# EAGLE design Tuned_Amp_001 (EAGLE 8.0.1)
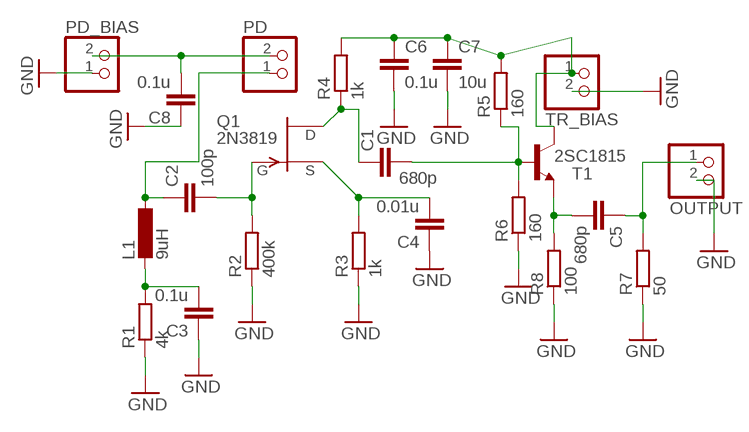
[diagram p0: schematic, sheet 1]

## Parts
C1  680p  C-EU025-024X044  [C025-024X044]
C2  100p  C-EU025-024X044  [C025-024X044]
C3  0.1u  C-EU025-024X044  [C025-024X044]
C4  0.01u  C-EU025-024X044  [C025-024X044]
C5  680p  C-EU025-024X044  [C025-024X044]
C6  0.1u  C-EU025-024X044  [C025-024X044]
C7  10u  C-EU025-024X044  [C025-024X044]
C8  0.1u  C-EU025-024X044  [C025-024X044]
L1  9uH  L-EU0207/10  [0207/10]
OUTPUT  JST_2PIN-SMT  [JST-PH-2-SMT]
PD  JST_2PIN-SMT  [JST-PH-2-SMT]
PD_BIAS  JST_2PIN-SMT  [JST-PH-2-SMT]
Q1  2N3819  [TO92]
R1  4k  R-EU_0207/10  [0207/10]
R2  400k  R-EU_0207/10  [0207/10]
R3  1k  R-EU_0207/10  [0207/10]
R4  1k  R-EU_0207/10  [0207/10]
R5  160  R-EU_0207/10  [0207/10]
R6  160  R-EU_0207/10  [0207/10]
R7  50  R-EU_0207/10  [0207/10]
R8  100  R-EU_0207/10  [0207/10]
T1  2SC1815  [TO92-ECB]
TR_BIAS  JST_2PIN-SMT  [JST-PH-2-SMT]

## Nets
GND: C3.1 C4.1 C6.2 C7.2 C8.1 OUTPUT.2 PD_BIAS.1 R1.1 R2.1 R3.1 R6.1 R7.1 R8.1 TR_BIAS.2
N$1: C2.2 Q1.2(G) R2.2
N$2: C3.2 L1.2 R1.2
N$3: C2.1 L1.1 PD.1
N$4: C6.1 C7.1 R4.2 R5.2 T1.C TR_BIAS.1
N$5: C1.1 Q1.1(D) R4.1
N$6: C1.2 R5.1 R6.2 T1.B
N$7: C4.2 Q1.3(S) R3.2
N$8: C8.2 PD.2 PD_BIAS.2
N$9: C5.2 R8.2 T1.E
N$10: C5.1 OUTPUT.1 R7.2

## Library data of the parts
C1-C8 = rcl:C-EU: CAPACITOR, European symbol
L1 = rcl:L-EU: INDUCTOR, European symbol
OUTPUT PD PD_BIAS TR_BIAS = adafruit:JST_2PIN: JST 2-Pin Connectors of various flavors
Q1 = transistor-fet:2N3819: N-Channel Junction FET
R1-R8 = rcl:R-EU_: RESISTOR, European symbol
T1 = transistor:2SC1815: NPN EPITAXIAL TRANSISTOR Source: TOSHIBA .. 2SC1815 1.pdf

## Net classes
0 default: width 0.305 mm, drill 0.508 mm, clearance 0.254 mm

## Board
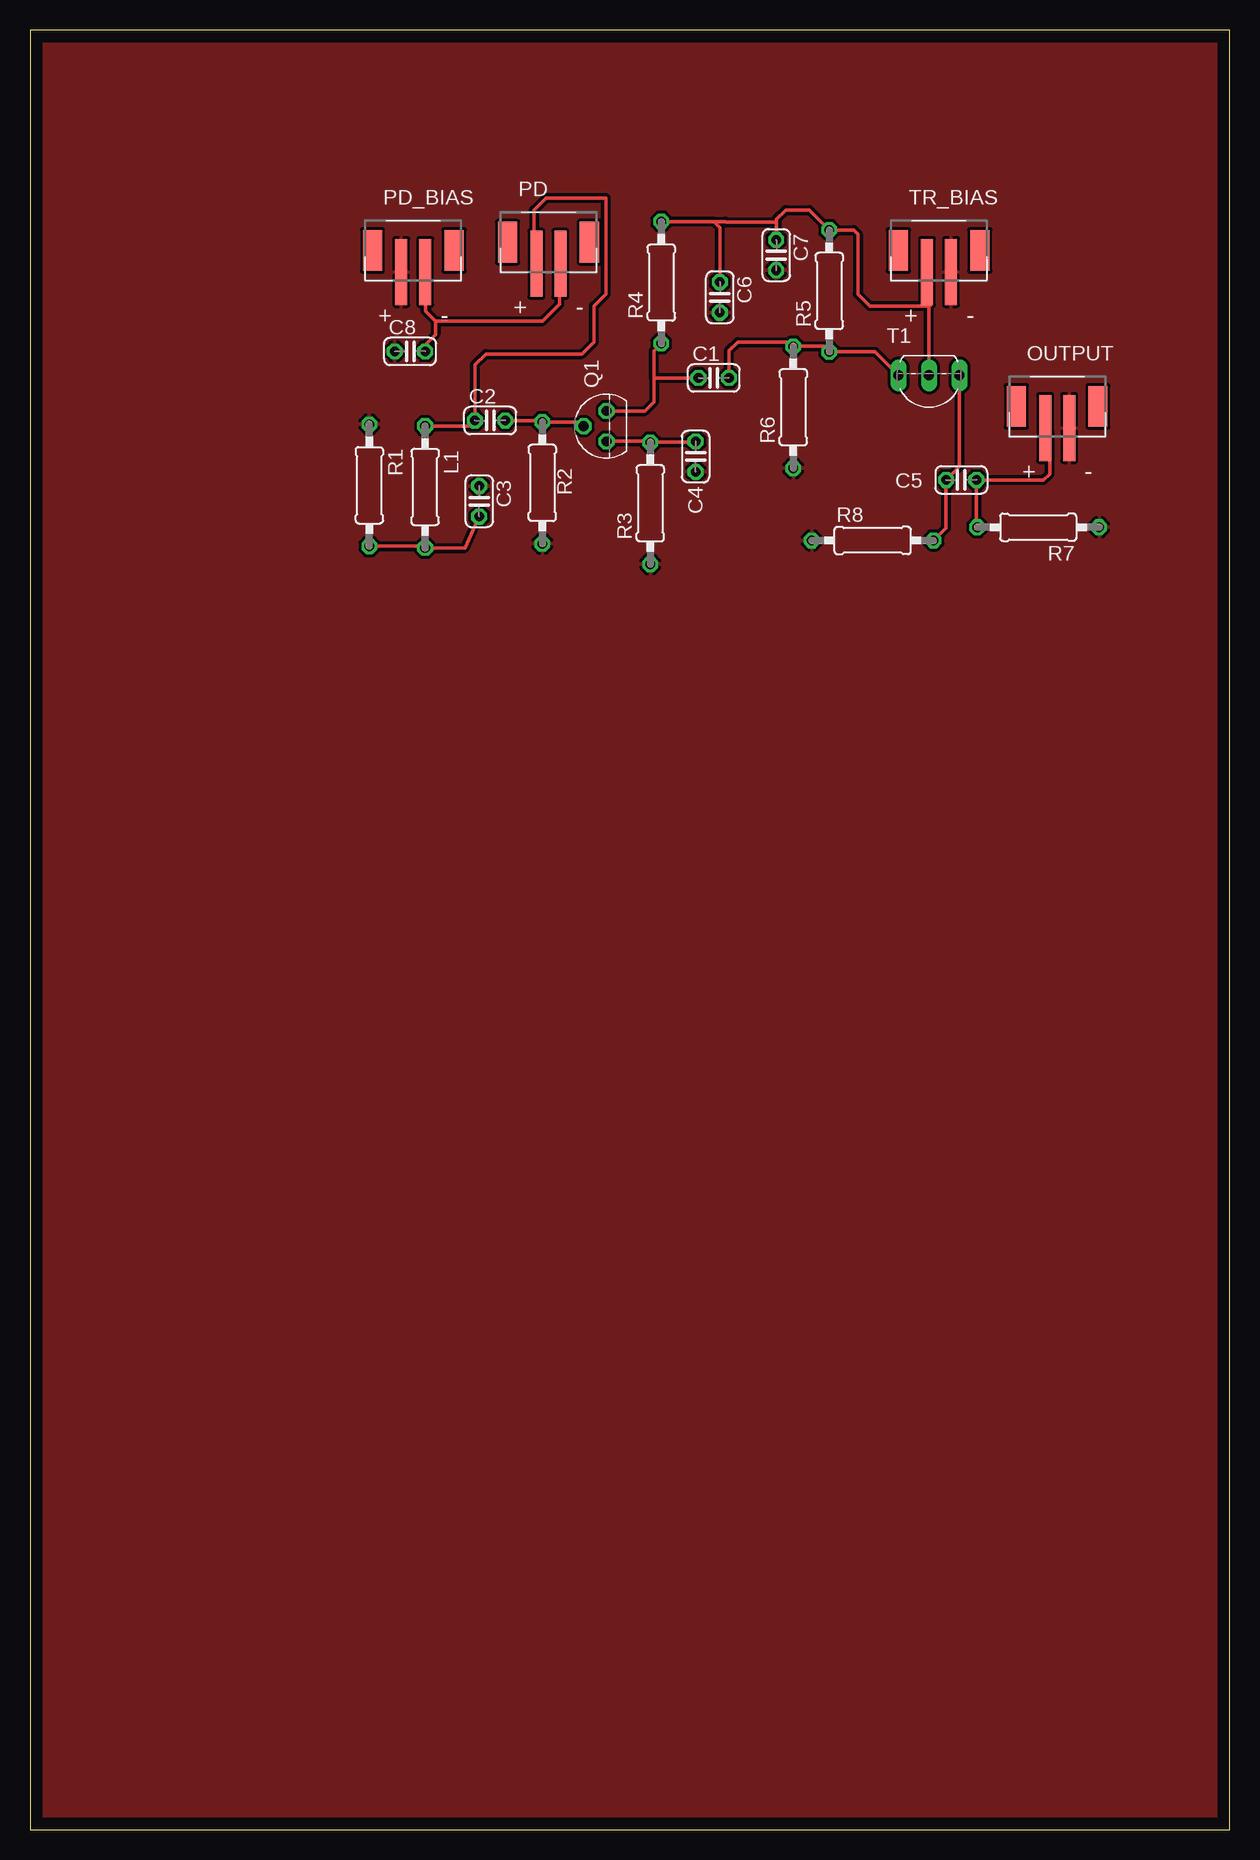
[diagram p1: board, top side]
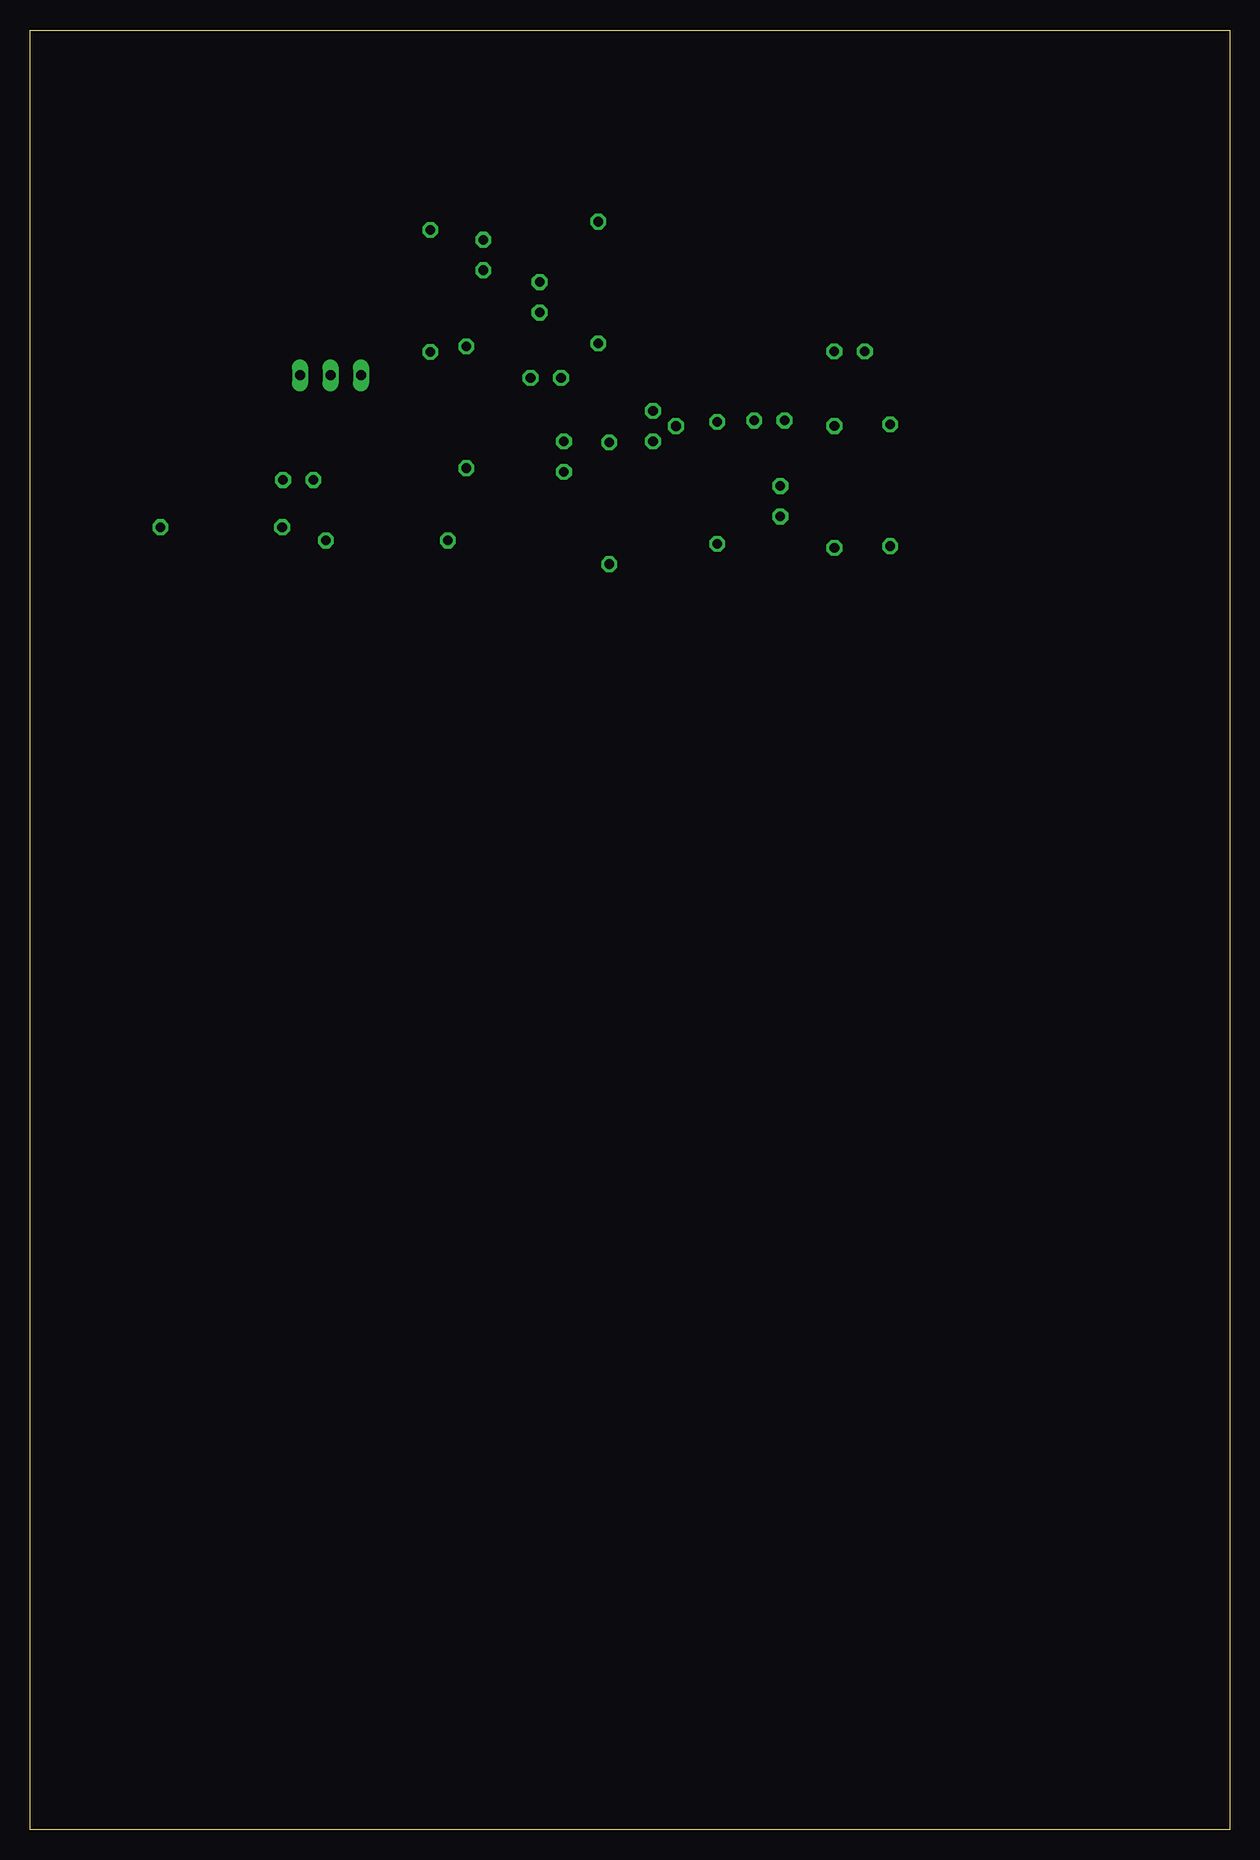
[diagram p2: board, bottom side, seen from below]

Size 100 x 150 mm. Coordinates in mm from the lower left corner, seen from the top.
Outline: 0,0 100,0 100,150 0,150 0,0
Copper layers (1*16): Top 0.035mm / dielectric 1.5mm / Bottom 0.035mm
Design rules "default": minimum track width 6mil, minimum drill 0.35mm, track to track 6mil, track to pad 6mil, pad to pad 6mil, via to via 6mil, smd to smd 6mil, copper to edge 40mil, drill to drill 6mil, minimum pad ring 10mil, minimum via ring 8mil, stop-mask expansion 4mil, vias tented up to drill 0mil, thermal gap 10mil

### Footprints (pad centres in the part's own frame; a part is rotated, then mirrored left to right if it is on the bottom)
C025-024X044 = drill 0.813 octagon: 1 -1.27,0; 2 1.27,0
0207/10 = drill 0.813 octagon: 1 -5.08,0; 2 5.08,0
JST-PH-2-SMT = smd 1 x 5.5: 1 -1,-1.8; 2 1,-1.8 | smd 1.6 x 3.4: NC1 -3.4,0; NC2 3.4,0
TO92 = drill 0.813 octagon: 1 1.27,0; 2 0,1.905; 3 -1.27,0
TO92-ECB = drill 0.813 long: B 2.54,0; C 0,0; E -2.54,0

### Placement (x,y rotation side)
C1  57,121 0 top
C2  38.36,117.45 0 top
C3  37.45,110.72 270 top
C4  55.49,114.44 90 top
C5  77.64,112.49 180 top
C6  57.51,127.72 270 top
C7  62.21,131.24 270 top
C8  31.68,123.21 0 top
L1  32.94,111.91 270 top
OUTPUT  85.63,118.62 0 top
PD  43.22,132.32 0 top
PD_BIAS  31.95,131.62 0 top
Q1  48.06,116.98 90 top
R1  28.29,112.05 270 top
R2  42.71,112.25 90 top
R3  51.71,110.55 90 top
R4  52.63,128.95 90 top
R5  66.63,128.25 90 top
R6  63.63,118.55 90 top
R7  84.05,108.55 180 top
R8  70.25,107.45 0 top
T1  74.94,121.22 180 top
TR_BIAS  75.79,131.62 0 top

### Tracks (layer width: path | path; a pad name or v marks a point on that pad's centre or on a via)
GND
  pour Top: -1,151 101,151 101,-1 -1,-1
N$1
  Top 0.305: C2.2 42.59,117.45 R2.2 45.8,117.33 Q1.2
N$2
  Top 0.305: C3.2 36.27,106.83 L1.2 32.8,106.97 R1.2
N$3
  Top 0.305: L1.1 36.63,116.99 C2.1 37.09,122.09 38,123 46,123 47,124 47,127 48,128 48,136 43,136 42,135 42,130.74 PD.1
N$4
  Top 0.305: 62.21,134 C7.1 | 62.21,134 62.21,134.21 63,135 64.96,135 R5.2 68.67,133.33 69,133 69,128 70,127 75,127 | 75,127 75,129.61 TR_BIAS.1 | T1.C 74.94,126.94 75,127 | 57,134.03 R4.2 | 57,134.03 57.97,134.03 58,134 62.21,134 | C6.1 57.51,133.52 57,134.03
  Bottom 0.305: 66.78,133.27 R5.2
N$5
  Top 0.305: Q1.1 51.25,118.25 52,119 52,121 | 52,121 52,123.24 R4.1 | C1.1 52,121
N$6
  Top 0.305: T1.B 70.45,123.17 R5.1 66.17,123.63 R6.2 63.26,124 59,124 58.27,123.27 C1.2
  Bottom 0.305: 63.98,123.22 63.7,123.5 R6.2 | 66.5,123.22 R5.1 66.78,122.94 | 72.36,121.26 T1.B
N$7
  Top 0.305: Q1.3 51.63,115.71 R3.2 55.41,115.63 C4.2
N$8
  Top 0.305: 33.81,125.73 33.81,124.61 32.97,123.77 32.97,123.22 C8.2 | 33.81,125.73 32.97,126.57 32.97,129.64 PD_BIAS.2 | 33.81,125.73 42.75,125.73 44.15,127.13 44.15,130.48 PD.2
N$9
  Top 0.305: T1.E 77.48,113.6 C5.2 76.37,108.49 R8.2
N$10
  Top 0.305: OUTPUT.1 85,116.45 85,113 84.49,112.49 C5.1 78.91,108.61 R7.2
